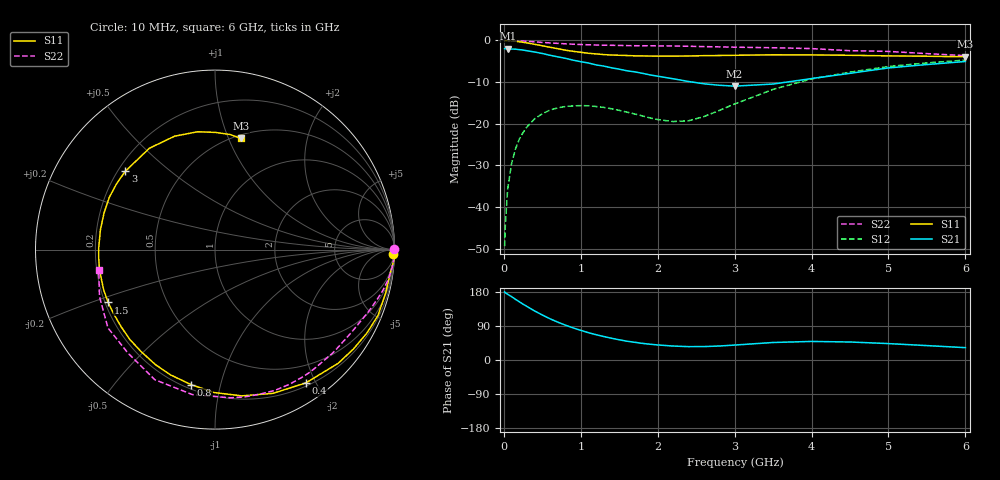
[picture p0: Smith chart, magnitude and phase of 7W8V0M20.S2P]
! Infineon Technologies  Discrete & RF Semiconductors
! BFS17W
! Si NPN RF Bipolar Junction Transistor in SOT323
! VCE = 8 V  IC = 0.2 mA
! Common Emitter S-Parameters:  August  1999
# GHz  S  MA  R  50
!  f  S11  S21  S12  S22
! GHz  MAG  ANG  MAG  ANG  MAG  ANG  MAG  ANG
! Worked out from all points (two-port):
!   36 points, 10 MHz to 6 GHz, reference 50 ohm
!   highest |S21| = -1.95 dB at 50 MHz (marker M1); lowest = -11.0 dB at 3 GHz (marker M2)
!   |S21| within 3 dB of the highest: start of sweep to 959.3 MHz
!   lowest |S11| = -3.9 dB at 6 GHz (marker M3), VSWR 4.50, Z = 26.6 + j55.4 ohm
!   |S11| at or under -10 dB: nowhere
!   |S22| runs from -3.6 to 0.0 dB; largest |S21 - S12| = 0.8
!   S11 on the Smith chart (normalised r, x): 10 MHz: 34, -72; 400 MHz: 0.24, -1.87; 800 MHz: 0.23, -0.81; 1.5 GHz: 0.21, -0.22; 3 GHz: 0.23, +0.36; 6 GHz: 0.53, +1.11
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0.01  0.9894 -1.3  0.796 179.6  0.0034 84.2  0.9999 0.2
0.02  0.9999 -3.0  0.798 177.5  0.0063 87.2  0.9989 -0.7
0.05  0.9856 -7.3  0.799 173.4  0.0165 87.6  0.998 -1.8
0.1  0.9813 -14.2  0.788 167.2  0.0331 81.6  0.9965 -3.7
0.15  0.9794 -22.1  0.787 160.3  0.0494 75.9  0.9923 -5.5
0.25  0.9495 -35.7  0.767 147.4  0.0785 67.8  0.9819 -9.0
0.4  0.8988 -55.7  0.727 129.4  0.1147 56.2  0.9619 -13.8
0.5  0.8638 -68.0  0.698 118.8  0.132 49.3  0.9469 -16.7
0.6  0.8286 -79.6  0.664 108.8  0.1461 43.5  0.9337 -19.4
0.8  0.7641 -100.0  0.611 92.0  0.1613 33.7  0.9108 -24.6
1.1  0.7014 -126.1  0.536 72.0  0.1645 23.2  0.8872 -31.9
1.5  0.6642 -153.7  0.452 53.3  0.145 17.3  0.8719 -41.9
1.8  0.6526 -170.9  0.404 43.9  0.1244 19.6  0.8641 -50.1
2.2  0.6479 170.3  0.347 36.8  0.1064 36.3  0.8576 -61.0
2.6  0.657 153.6  0.302 35.4  0.122 60.0  0.8435 -72.6
3  0.6637 138.9  0.283 39.4  0.1729 71.6  0.8304 -83.9
3.5  0.6727 122.9  0.3 46.2  0.2588 72.4  0.8177 -98.8
4  0.6707 109.6  0.349 49.0  0.3455 66.3  0.7986 -114.8
4.5  0.6637 98.4  0.403 47.5  0.4166 58.5  0.7535 -130.0
5  0.653 89.8  0.468 43.3  0.4867 50.8  0.739 -143.8
5.5  0.6467 82.6  0.514 38.0  0.5378 43.1  0.6947 -157.9
6  0.6364 77.0  0.559 32.6  0.5819 36.1  0.6575 -170.2
